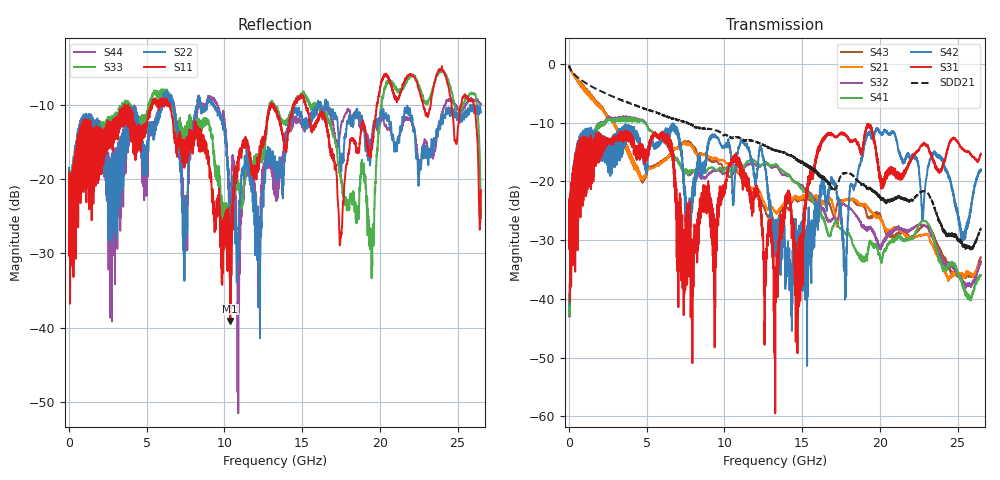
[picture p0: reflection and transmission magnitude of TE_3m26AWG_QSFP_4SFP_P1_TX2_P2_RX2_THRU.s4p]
!Agilent Technologies,N5222A,MY51421691,A.10.00.00
!Agilent N5222A: A.10.00.00
!Date: Friday, January 30, 2015 12:33:12
!Correction: S11(Full 4 Port(1,2,3,4))
!S12(Full 4 Port(1,2,3,4))
!S13(Full 4 Port(1,2,3,4))
!S14(Full 4 Port(1,2,3,4))
!S21(Full 4 Port(1,2,3,4))
!S22(Full 4 Port(1,2,3,4))
!S23(Full 4 Port(1,2,3,4))
!S24(Full 4 Port(1,2,3,4))
!S31(Full 4 Port(1,2,3,4))
!S32(Full 4 Port(1,2,3,4))
!S33(Full 4 Port(1,2,3,4))
!S34(Full 4 Port(1,2,3,4))
!S41(Full 4 Port(1,2,3,4))
!S42(Full 4 Port(1,2,3,4))
!S43(Full 4 Port(1,2,3,4))
!S44(Full 4 Port(1,2,3,4))
!S4P File: Measurements: <S11,S12,S13,S14>,
!<S21,S22,S23,S24>,
!<S31,S32,S33,S34>,
!<S41,S42,S43,S44>:
# Hz S  dB  R 50.0
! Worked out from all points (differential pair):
!   2650 points, 10 MHz to 26.5 GHz, reference 50 ohm
!   strongest paths, dB at 10 MHz, 6.63 GHz, 13.26 GHz, 19.88 GHz, 26.5 GHz:
!     S31: -24.7, -15.6, -42.4, -17.4, -15.3
!     S42: -24.8, -11.1, -30.4, -11.2, -17.9
!     S41: -39.9, -15.1, -17.1, -31.7, -36.0
!     S32: -40.0, -15.4, -17.5, -30.4, -33.7
!     S21: -0.4, -14.9, -25.0, -25.9, -34.0
!     S43: -0.4, -15.1, -27.1, -25.4, -32.9
!   taken as a pair (ports 1,3 in; 2,4 out), SDD21 dB: -0.3, -9.3, -14.7, -22.2, -28.2
!   lowest |S11| = -39.1 dB at 10.38 GHz (marker M1), VSWR 1.02, Z = 49.4 + j0.904 ohm
!   |S11| at or under -10 dB: start of sweep to 3.58 GHz; 6.484 GHz to 12.98 GHz (6.496 GHz wide, 66.8 % of centre); 15.24 GHz to 19.8 GHz (4.559 GHz wide, 26 % of centre)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
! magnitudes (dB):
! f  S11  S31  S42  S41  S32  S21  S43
! 10 MHz  -19.1  -24.7  -24.8  -39.9  -40.0  -0.4  -0.4
! 1.96 GHz  -13.8  -12.7  -12.0  -10.9  -10.7  -7.1  -7.0
! 7.92 GHz  -14.9  -34.2  -22.4  -18.0  -18.3  -14.1  -13.8
! 10.38 GHz  -39.1  -17.4  -14.7  -18.3  -17.2  -17.0  -19.2
! 13.3 GHz  -11.0  -36.0  -28.9  -17.1  -17.4  -25.2  -27.4
! 16.61 GHz  -13.4  -12.2  -23.8  -28.3  -26.3  -23.3  -23.5
! 26.5 GHz  -21.5  -15.3  -17.9  -36.0  -33.7  -34.0  -32.9
